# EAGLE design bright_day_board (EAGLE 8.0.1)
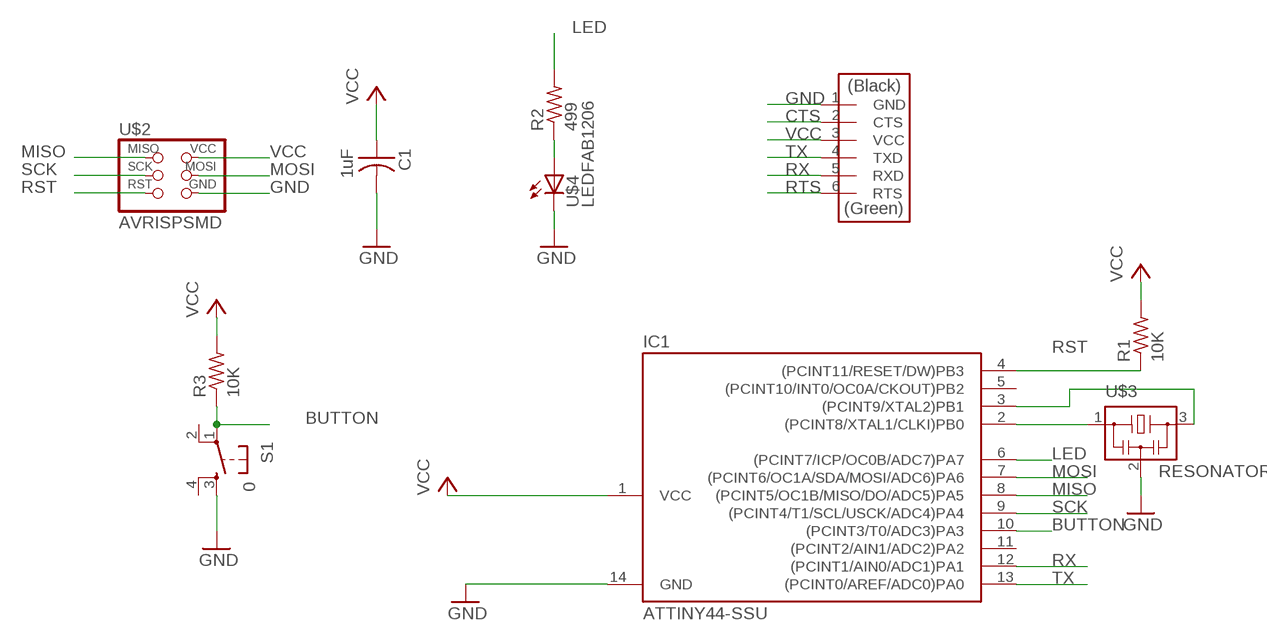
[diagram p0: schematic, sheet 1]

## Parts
C1  1uF  CAP-US1206  [C1206]
IC1  ATTINY44-SSU  [SOIC14]
R1  10K  RES-US1206  [R1206]
R2  499  RES-US1206FAB  [R1206FAB]
R3  10K  RES-US1206  [R1206]
S1  0  6MM_SWITCH6MM_SWITCH  [6MM_SWITCH]
U$1  FTDI-SMD-HEADER  [1X06SMD]
U$2  AVRISPSMD  [2X03SMD]
U$3  RESONATOR  [EFOBM]
U$4  LEDFAB1206  [LED1206FAB]

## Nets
BUTTON: IC1.10((PCINT3/T0/ADC3)PA3) R3.1 S1.1(P)
CTS: U$1.2(CTS)
GND: C1.2 IC1.14(GND) S1.3(S) U$1.1(GND) U$2.6(GND) U$3.2 U$4.2(C)
LED: IC1.6((PCINT7/ICP/OC0B/ADC7)PA7) R2.2
MISO: IC1.8((PCINT5/OC1B/MISO/DO/ADC5)PA5) U$2.1(MISO)
MOSI: IC1.7((PCINT6/OC1A/SDA/MOSI/ADC6)PA6) U$2.4(MOSI)
N$4: IC1.3((PCINT9/XTAL2)PB1) U$3.3
N$5: IC1.2((PCINT8/XTAL1/CLKI)PB0) U$3.1
N$6: R2.1 U$4.1(A)
RST: IC1.4((PCINT11/RESET/DW)PB3) R1.1 U$2.5(RST)
RTS: U$1.6(RTS)
RX: IC1.12((PCINT1/AIN0/ADC1)PA1) U$1.5(RXD)
SCK: IC1.9((PCINT4/T1/SCL/USCK/ADC4)PA4) U$2.3(SCK)
TX: IC1.13((PCINT0/AREF/ADC0)PA0) U$1.4(TXD)
VCC: C1.1 IC1.1(VCC) R1.2 R3.2 U$1.3(VCC) U$2.2(VCC)
Unconnected: IC1.5((PCINT10/INT0/OC0A/CKOUT)PB2) IC1.11((PCINT2/AIN1/ADC2)PA2) S1.2(P1) S1.4(S1)

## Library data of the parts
C1 = fab:CAP-US
IC1 = fab:ATTINY44
R1-R3 = fab:RES-US: Resistor (US Symbol)
S1 = fab:6MM_SWITCH: OMRON SWITCH
U$1 = fab:FTDI-SMD-HEADER
U$2 = fab:AVRISP
U$3 = fab:RESONATOR
U$4 = fab:LED: LED

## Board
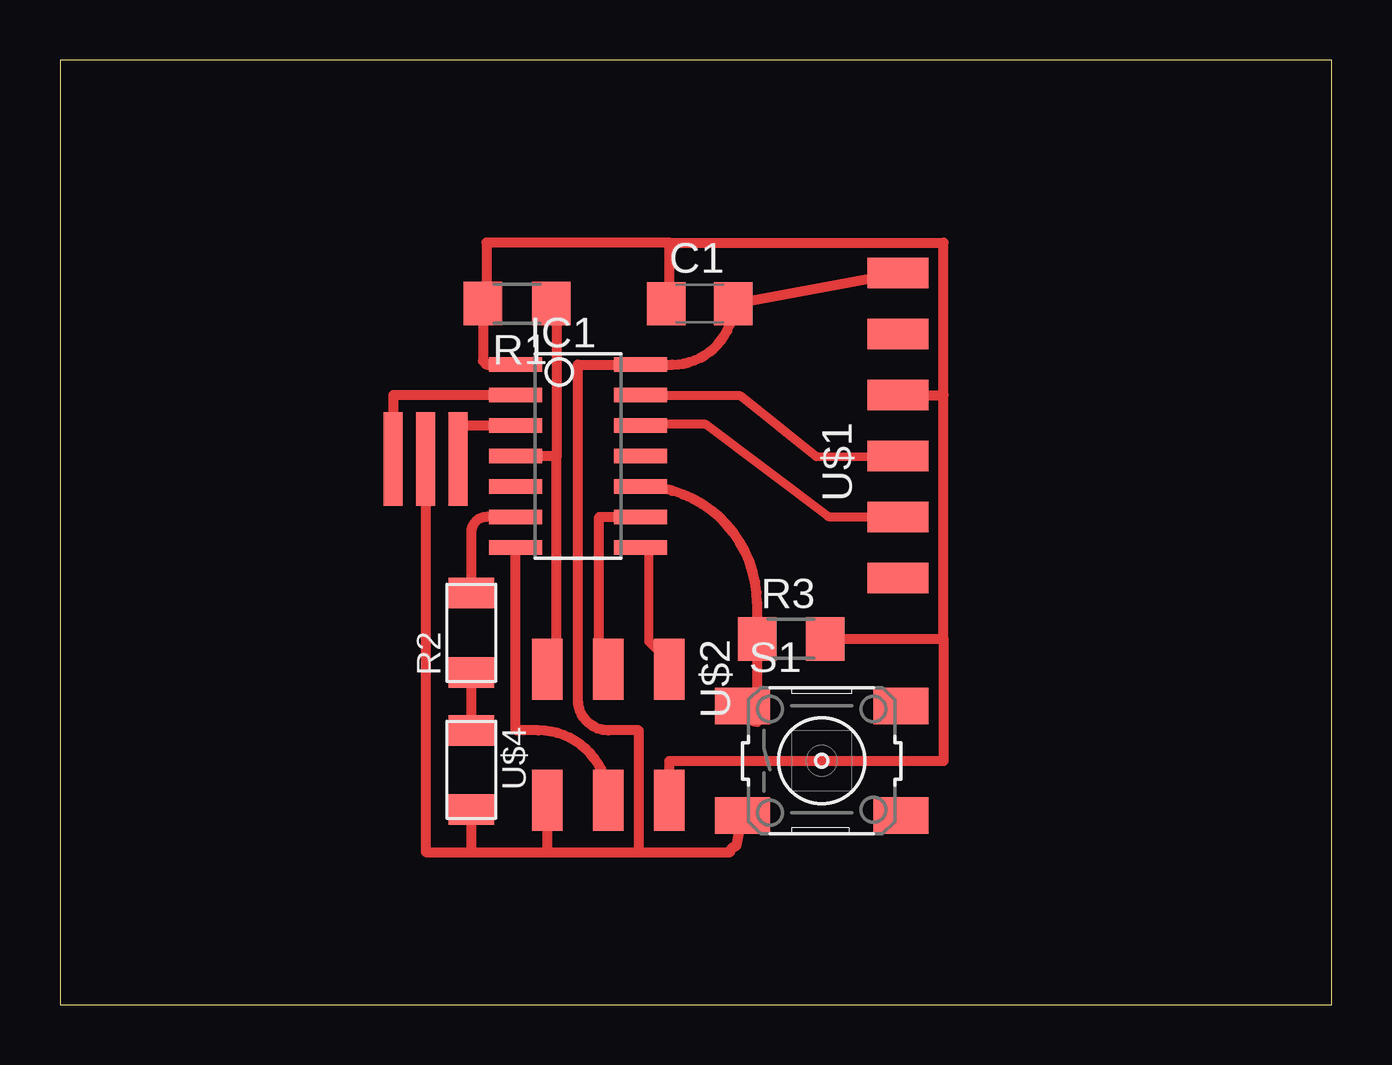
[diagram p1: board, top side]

Size 53.01 x 39.36 mm. Coordinates in mm from the lower left corner, seen from the top.
Outline: 0,0 53.01,0 53.01,39.36 0,39.36 0,0
Copper layers (1*16): Top 0.035mm / dielectric 1.5mm / Bottom 0.035mm
Design rules "default *": minimum track width 15mil, minimum drill 24mil, track to track 16mil, track to pad 16mil, pad to pad 16mil, via to via 16mil, smd to smd 16mil, copper to edge 40mil, drill to drill 8mil, minimum pad ring 10mil, minimum via ring 8mil, stop-mask expansion 4mil, vias tented up to drill 0mil, thermal gap 10mil

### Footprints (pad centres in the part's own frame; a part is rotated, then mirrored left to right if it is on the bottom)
C1206 = smd 1.6 x 1.8: 1 -1.4,0; 2 1.4,0
SOIC14 = smd 0.61 x 2.21: 1 -3.81,-2.603; 2 -2.54,-2.603; 3 -1.27,-2.603; 4 0,-2.603; 5 1.27,-2.603; 6 2.54,-2.603; 7 3.81,-2.603; 8 3.81,2.603; 9 2.54,2.603; 10 1.27,2.603; 11 0,2.603; 12 -1.27,2.603; 13 -2.54,2.603; 14 -3.81,2.603
R1206 = smd 1.6 x 1.803: 1 -1.422,0; 2 1.422,0
R1206FAB = smd 1.27 x 1.905: 1 -1.651,0; 2 1.651,0
6MM_SWITCH = smd 2.286 x 1.524: 1 -3.302,2.286; 2 3.302,2.286; 3 -3.302,-2.286; 4 3.302,-2.286
1X06SMD = smd 2.54 x 1.27: 1 0,6.35; 2 0,3.81; 3 0,1.27; 4 0,-1.27; 5 0,-3.81; 6 0,-6.35
2X03SMD = smd 2.54 x 1.27: 1 -2.54,2.54; 2 2.92,2.54; 3 -2.54,0; 4 2.92,0; 5 -2.54,-2.54; 6 2.92,-2.54
EFOBM = smd 0.8 x 3.9: 1 -1.35,0; 2 0,0; 3 1.35,0
LED1206FAB = smd 1.27 x 1.905: 1 -1.651,0; 2 1.651,0

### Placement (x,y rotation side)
C1  26.67,29.21 0 top
IC1  21.59,22.86 270 top
R1  19.05,29.21 180 top
R2  17.15,15.49 90 top
R3  30.48,15.24 0 top
S1  31.75,10.16 0 top
U$1  34.92,24.13 0 top
U$2  22.86,11.43 270 top
U$3  15.24,22.73 0 top
U$4  17.15,9.78 270 top

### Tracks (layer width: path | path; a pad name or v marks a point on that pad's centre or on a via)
BUTTON
  Top 0.406: IC1.10 arc-90 29.06,16.73 R3.1 29.06,11.79 arc-90 S1.1
GND
  Top 0.406: 20.32,6.35 U$2.6 | 20.32,6.35 24.13,6.35 | 24.13,6.35 24.13,11.43 22.86,11.43 arc-90 21.59,12.7 21.59,26.67 IC1.14 25.53,26.67 arc90 C1.2 U$1.1 | 17.15,6.35 20.32,6.35 | 24.13,6.35 27.94,6.35 arc-90 28.19,6.6 S1.3 | U$4.2 17.15,6.35 | U$3.2 15.24,6.35 17.15,6.35
LED
  Top 0.406: IC1.6 17.78,20.32 arc90 17.15,19.68 R2.2
MISO
  Top 0.381: IC1.8 24.55,19.06 24.55,15.13 25.34,14.34 U$2.1
MOSI
  Top 0.406: U$2.4 arc90 19.94,11.43 19.05,11.43 arc-90 18.99,11.49 IC1.7
N$4
  Top 0.381: 18.64,24.18 IC1.3
  Top 0.406: IC1.3 16.59,24.13 U$3.3
N$5
  Top 0.381: 18.64,25.36 IC1.2
  Top 0.406: IC1.2 13.89,25.4 U$3.1
N$6
  Top 0.406: R2.1 U$4.1
RST
  Top 0.406: 20.95,29.21 R1.1 20.7,29.11 20.7,22.86 | 20.7,22.86 IC1.4 | U$2.5 20.7,13.84 20.7,22.86
RX
  Top 0.381: IC1.12 24.55,24.18 26.91,24.18 32.03,20.33 U$1.5
SCK
  Top 0.406: IC1.9 22.48,20.32 22.48,14.48 arc90 U$2.3
TX
  Top 0.381: IC1.13 24.55,25.36 28.36,25.36 31.52,22.84 U$1.4
VCC
  Top 0.406: U$1.3 36.83,25.4 | 36.83,25.4 36.83,31.75 25.4,31.75 | 25.4,31.75 17.78,31.75 17.78,29.36 R1.2 17.63,26.82 17.78,26.67 IC1.1 | C1.1 25.4,29.21 25.4,31.75 | 36.83,15.24 36.83,10.16 25.4,10.16 U$2.2 | 36.83,15.24 36.83,25.4 | R3.2 36.83,15.24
